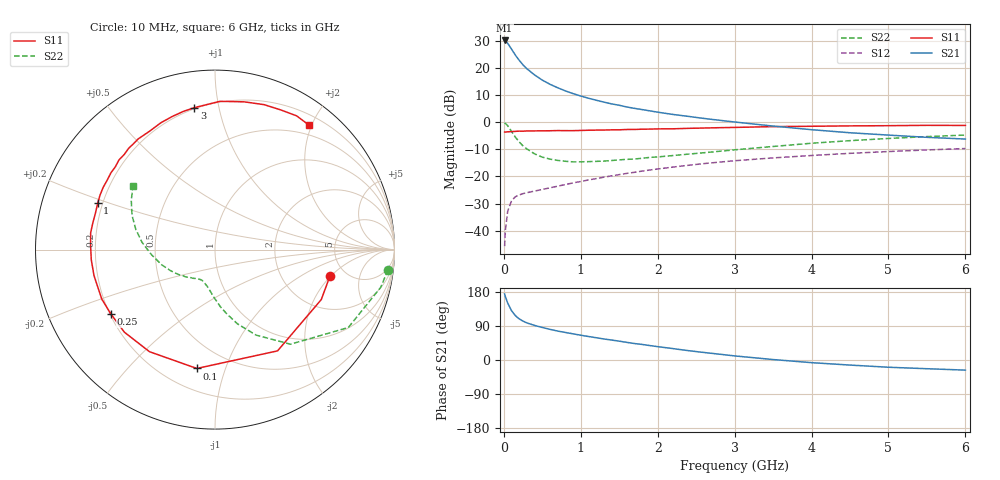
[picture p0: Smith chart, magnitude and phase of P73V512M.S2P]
! SIEMENS Small Signal Semiconductors
! BFP196
! Si NPN RF Bipolar Junction Transistor in SOT143
! VCE = 3.5 V  IC = 12 mA
! Common Emitter S-Parameters:  May  1996
# GHz  S  MA  R  50
!  f  S11  S21  S12  S22
! GHz  MAG  ANG  MAG  ANG  MAG  ANG  MAG  ANG
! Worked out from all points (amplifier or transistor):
!   36 points, 10 MHz to 6 GHz, reference 50 ohm
!   highest |S21| = 30.1 dB at 10 MHz (marker M1)
!   |S21| within 3 dB of that: start of sweep to 95.82 MHz
!   unconditionally stable (mu >= 1): 814.8 MHz to 3.263 GHz
!   at 250 MHz: K = 0.45, MSG = 23.7 dB, |S12| = -26.3 dB
!   at 1.4 GHz: K = 1.13, MAG = 11.1 dB, |S12| = -19.8 dB
!   at 6 GHz: K = 0.98, MSG = 1.7 dB, |S12| = -9.7 dB
!   S11 on the Smith chart (normalised r, x): 10 MHz: 3.77, -1.95; 100 MHz: 0.33, -0.80; 250 MHz: 0.20, -0.27; 1 GHz: 0.18, +0.18; 3 GHz: 0.19, +0.85; 6 GHz: 0.35, +1.96
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0.01  0.6573 -12.9  31.91 174.4  0.0052 85.9  0.9699 -6.7
0.02  0.6543 -25.2  30.97 167.1  0.0102 77.2  0.9472 -12.8
0.05  0.6632 -58.3  28.27 150.5  0.0229 64.9  0.8603 -30.3
0.1  0.6699 -98.7  22.13 130.2  0.0357 49.3  0.6743 -51.4
0.15  0.6759 -122.7  17.11 117.0  0.0423 40.9  0.5289 -64.3
0.2  0.6832 -137.7  13.74 108.5  0.0456 37.2  0.4318 -73.2
0.25  0.682 -148.3  11.29 102.5  0.0483 35.4  0.3637 -79.6
0.3  0.6885 -156.4  9.614 97.9  0.0502 35.4  0.3209 -84.5
0.4  0.6895 -167.9  7.388 91.2  0.0538 35.9  0.2602 -92.2
0.5  0.6917 -175.3  5.937 85.8  0.0576 37.1  0.2265 -97.8
0.6  0.6937 177.9  4.975 80.9  0.0617 39.1  0.2085 -102.2
0.7  0.6991 172.3  4.296 76.3  0.0662 40.5  0.1973 -106.4
0.8  0.6967 167.6  3.758 72.7  0.0709 42.1  0.1903 -110.0
1  0.7027 158.4  3.023 65.4  0.0807 44.4  0.1856 -115.6
1.1  0.709 154.6  2.757 62.0  0.0861 45.3  0.1873 -118.4
1.6  0.732 137.0  1.899 46.5  0.1139 46.0  0.2063 -130.6
2.2  0.7537 118.9  1.384 30.0  0.1488 42.9  0.2426 -144.4
3  0.799 98.3  1.006 10.8  0.1946 35.3  0.309 -164.1
3.5  0.8266 88.1  0.846 1.2  0.2195 29.8  0.3563 -175.7
4.5  0.8527 71.3  0.637 -13.4  0.2664 18.8  0.4562 165.5
5.5  0.873 58.6  0.525 -23.0  0.3075 7.6  0.5414 149.5
6  0.8691 52.9  0.488 -26.7  0.3266 1.7  0.5781 142.2
